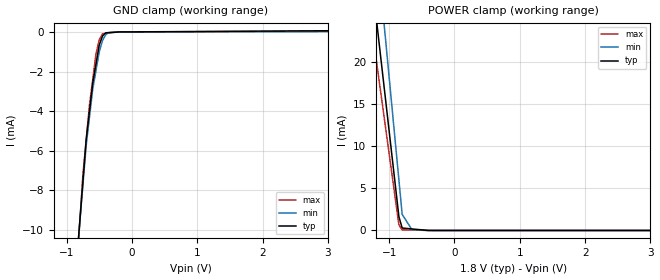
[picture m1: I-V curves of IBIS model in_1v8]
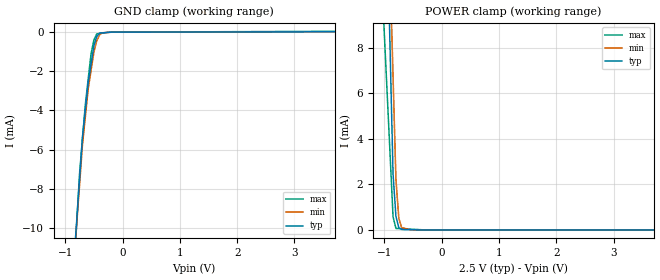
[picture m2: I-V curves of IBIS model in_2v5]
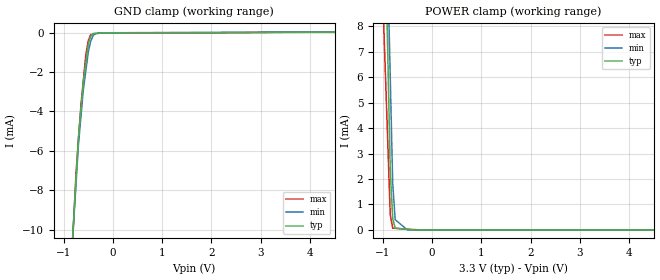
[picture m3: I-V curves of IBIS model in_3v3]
[IBIS Ver]   3.2
[Comment Char] |_char
[File Name]   tlv320aic25i.ibs
[File Rev]   3.0
[Source]
| This model file was created by Teraspeed Consulting Group LLC
| (http://www.teraspeed.com/).
[Date]   10-06-2007
[Notes]   Quality Check of this IBIS model: Model Passes IBIS Check
   Model parses into ICX IS. Simulation done with Hyperlynx.
   1. MIN TYP MAX information is based on Temprature and Voltage
   characteristics only.
[Disclaimer]
| This model is designed as an aid for customers of Texas Instruments.
| TI and its licensors and suppliers make no warranties, either expressed
| or implied, with respect to this  model, including the warranties of
| merchantability or fitness for a particular purpose.
| The model is provided solely on an "as is" basis. The entire risk as to
| its quality and performance is with the customer.
[Copyright]
| (C) Copyright 2008 Texas Instruments Incorporated. All rights reserved.
[Component] TLV320AIC25I
[Manufacturer] TI
[Package]
| variable   typ   min   max
R_pkg  1.8006E-02  1.8006E-02  1.8006E-02
L_pkg  2.1607E-09  2.1607E-09  2.1607E-09
C_pkg  6.0021E-13  6.0021E-13  6.0021E-13
[Pin] signal_name  model_name  R_pin  L_pin C_pin
1   HDSI-   analog   1.89E-02  2.26E-09  6.29E-13
2   HDSI+   analog   1.80E-02  2.16E-09  6.01E-13
3   HDSO-   analog   1.72E-02  2.06E-09  5.73E-13
4   HDSO+   analog   1.64E-02  1.97E-09  5.47E-13
5   AVDD2   POWER   1.56E-02  1.87E-09  5.21E-13
6   AVSS2   GND   1.49E-02  1.78E-09  4.96E-13
7   TESTP   analog   1.49E-02  1.78E-09  4.96E-13
8   NC   NC   1.56E-02  1.87E-09  5.21E-13
9   _PWRDN   in   1.64E-02  1.97E-09  5.47E-13
10   SDA   out_io_od 1.72E-02  2.06E-09  5.73E-13
11   SCL   in   1.80E-02  2.16E-09  6.01E-13
12   IOVDD   POWER   1.89E-02  2.26E-09  6.29E-13
13   IOVSS   GND   1.89E-02  2.26E-09  6.29E-13
14   FSD   out   1.80E-02  2.16E-09  6.01E-13
15   DVDD   POWER   1.72E-02  2.06E-09  5.73E-13
16   DVSS   GND   1.64E-02  1.97E-09  5.47E-13
17   DOUT   out   1.56E-02  1.87E-09  5.21E-13
18   DIN   in   1.49E-02  1.78E-09  4.96E-13
19   FS   out_io   1.49E-02  1.78E-09  4.96E-13
20   SCLK   out_io   1.56E-02  1.87E-09  5.21E-13
21   M/S   in   1.64E-02  1.97E-09  5.47E-13
22   MCLK   in   1.72E-02  2.06E-09  5.73E-13
23   _RESET   in   1.80E-02  2.16E-09  6.01E-13
24   VSS   GND   1.89E-02  2.26E-09  6.29E-13
25   DRVSS1   GND   1.89E-02  2.26E-09  6.29E-13
26   SPKO+   analog   1.80E-02  2.16E-09  6.01E-13
27   DRVDD   POWER   1.72E-02  2.06E-09  5.73E-13
28   SPKO-   analog   1.64E-02  1.97E-09  5.47E-13
29   DRVSS2   GND   1.56E-02  1.87E-09  5.21E-13
30   CIDI-   analog   1.49E-02  1.78E-09  4.96E-13
31   CIDI+   analog   1.49E-02  1.78E-09  4.96E-13
32   AVSS1   GND   1.56E-02  1.87E-09  5.21E-13
33   AVDD1   POWER   1.64E-02  1.97E-09  5.47E-13
34   MICI-   analog   1.72E-02  2.06E-09  5.73E-13
35   MICI+   analog   1.80E-02  2.16E-09  6.01E-13
36   MICBIAS   analog   1.89E-02  2.26E-09  6.29E-13
37   LCDAC   analog   1.89E-02  2.26E-09  6.29E-13
38   HNSO-   analog   1.80E-02  2.16E-09  6.01E-13
39   HNSO+   analog   1.72E-02  2.06E-09  5.73E-13
40   HNSI-   analog   1.64E-02  1.97E-09  5.47E-13
41   HNSI+   analog   1.56E-02  1.87E-09  5.21E-13
42   AVDD   POWER   1.49E-02  1.78E-09  4.96E-13
43   AVSS   GND   1.49E-02  1.78E-09  4.96E-13
44   LINEI+   analog   1.56E-02  1.87E-09  5.21E-13
45   LINEI-   analog   1.64E-02  1.97E-09  5.47E-13
46   LINEO-   analog   1.72E-02  2.06E-09  5.73E-13
47   LINEO+   analog   1.80E-02  2.16E-09  6.01E-13
48   NC   NC   1.89E-02  2.26E-09  6.29E-13
[Model Selector] in
in_1v8   input IOVDD=1.8V
in_2v5   input IOVDD=2.5V
in_3v3   input IOVDD=3.3V
[Model Selector] out
out_1v8  output IOVDD=1.8V
out_2v5  output IOVDD=2.5V
out_3v3  output IOVDD=3.3V
[Model Selector] out_io
io_1v8   io output IOVDD=1.8V
io_2v5   io output IOVDD=2.5V
io_3v3   io output IOVDD=3.3V
[Model Selector] out_io_od
od_1v8   open drain io IOVDD=1.8V
od_2v5   open drain io IOVDD=2.5V
od_3v3   open drain io IOVDD=3.3V
[Model] analog
Model_type Terminator
C_comp  0pF 0pF 0pF
| variable typ   min   max
[Voltage Range]   3.30000V  3.00000V  3.60000V
[POWER Clamp Reference]  3.30000V  3.00000V  3.60000V
[GND Clamp Reference]   0.00000V  0.00000V  0.00000V
[Temperature Range]   25   85   -40
| Models and submodels in the file (13): analog (Terminator), in_1v8 (Input), in_2v5 (Input), in_3v3 (Input), io_1v8 (I/O), io_2v5 (I/O), io_3v3 (I/O), od_1v8 (I/O_open_drain), od_2v5 (I/O_open_drain), od_3v3 (I/O_open_drain), out_1v8 (Output), out_2v5 (Output), out_3v3 (Output)
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[Model] in_1v8
Model_type Input
Vinl = 540.000mV
Vinh = 1.26000V
C_comp 865.00fF 865.00fF 865.00fF
| variable typ   min   max
[Voltage Range] 1.80000V 1.65000V 1.95000V
[POWER Clamp Reference] 1.80000V 1.65000V 1.95000V
[GND Clamp Reference] 0.00000V 0.00000V 0.00000V
[Temperature Range]   25   85   -40
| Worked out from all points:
|   GND clamp passes 1 mA (typ) near -0.52 V on its own axis
|   POWER clamp passes 1 mA (typ) near -0.83 V on its own axis
[GND Clamp]
-1.8V     -51.84mA   -49.48mA   -60.21mA
-750mV    -7.544mA   -7.715mA   -7.191mA
-700mV    -5.435mA   -5.726mA   -5.445mA
-650mV    -4.01mA    -4.308mA   -3.7mA
-600mV    -2.585mA   -2.89mA    -2.403mA
-550mV    -1.618mA   -1.944mA   -1.105mA
-500mV    -651.4uA   -998.2uA   -396.8uA
-450mV    -202.3uA   -430uA     -89.27uA
-400mV    -42.24uA   -132.6uA   -69.57uA
-350mV    -31.55uA   -30.96uA   -49.87uA
-175mV    1.006uA    -1.033uA   -9.754nA
3.6V      72.76uA    21.19uA    45.99uA
[POWER Clamp]
-1.8V     66.17mA    83.43mA    54.33mA
-1V       11.83mA    18.22mA    9.136mA
-950mV    8.432mA    14.15mA    6.311mA
-850mV    1.64mA     5.994mA    661.3uA
-800mV    291.4uA    1.919mA    76.17uA
-650mV    182.1uA    82.36uA    52.12uA
-600mV    145.7uA    64.06uA    44.1uA
-550mV    109.3uA    45.76uA    36.08uA
-475mV    54.63uA    22.88uA    24.05uA
-400mV    0A         0A         12.03uA
-275mV    0A         0A         0A
3.6V      0A         0A         0A
[Model] in_2v5
Model_type Input
Vinl = 750.000mV
Vinh = 1.75000V
C_comp 865.00fF 865.00fF 865.00fF
| variable typ   min   max
[Voltage Range] 2.50000V 2.25000V 2.75000V
[POWER Clamp Reference] 2.50000V 2.25000V 2.75000V
[GND Clamp Reference] 0.00000V 0.00000V 0.00000V
[Temperature Range]   25   85   -40
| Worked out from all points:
|   GND clamp passes 1 mA (typ) near -0.52 V on its own axis
|   POWER clamp passes 1 mA (typ) near -0.81 V on its own axis
[GND Clamp]
-2.5V     -81.75mA   -78.51mA   -95.22mA
-750mV    -7.485mA   -7.776mA   -7.19mA
-700mV    -5.363mA   -5.755mA   -5.442mA
-650mV    -3.969mA   -4.33mA    -3.694mA
-600mV    -2.576mA   -2.904mA   -2.397mA
-550mV    -1.626mA   -1.958mA   -1.1mA
-500mV    -676.1uA   -1.011mA   -393.6uA
-450mV    -219uA     -439.1uA   -88.29uA
-400mV    -47.76uA   -136.8uA   -68.84uA
-350mV    -36.13uA   -32.34uA   -49.39uA
-175mV    -1.107uA   -1.209uA   -232.2nA
5V        25.05uA    25.91uA    55.27uA
[POWER Clamp]
-2.5V     176.6mA    155mA      87.56mA
-1.05V    23.55mA    24.69mA    11.12mA
-850mV    2.446mA    6.718mA    573.1uA
-800mV    592.9uA    2.224mA    67.58uA
-750mV    103.1uA    517.3uA    61.15uA
-700mV    22.08uA    104.5uA    54.71uA
-550mV    12.62uA    10.89uA    35.4uA
-200mV    0A         0A         0A
5V        0A         0A         0A
[Model] in_3v3
Model_type Input
Vinl = 990.000mV
Vinh = 2.31000V
C_comp 865.00fF 865.00fF 865.00fF
| variable typ   min   max
[Voltage Range] 3.30000V 3.00000V 3.60000V
[POWER Clamp Reference] 3.30000V 3.00000V 3.60000V
[GND Clamp Reference] 0.00000V 0.00000V 0.00000V
[Temperature Range]   25   85   -40
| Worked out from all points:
|   GND clamp passes 1 mA (typ) near -0.52 V on its own axis
|   POWER clamp passes 1 mA (typ) near -0.81 V on its own axis
[GND Clamp]
-3.3V     -117.1mA   -110.4mA   -136.1mA
-750mV    -7.458mA   -7.71mA    -7.174mA
-700mV    -5.309mA   -5.696mA   -5.434mA
-650mV    -3.884mA   -4.286mA   -3.693mA
-600mV    -2.46mA    -2.876mA   -2.4mA
-550mV    -1.522mA   -1.931mA   -1.106mA
-500mV    -583uA     -986.8uA   -398.9uA
-450mV    -174uA     -421.8uA   -90.18uA
-400mV    -35.63uA   -128.7uA   -70.3uA
-350mV    -26.99uA   -29.92uA   -50.41uA
-175mV    -1.051uA   -656.6nA   -701.8nA
6.6V      61.64uA    70.47uA    89.11uA
[POWER Clamp]
-3.3V     226.6mA    210.1mA    138.5mA
-1.1V     25.2mA     26.83mA    14.67mA
-850mV    2.316mA    6.004mA    595.1uA
-800mV    453.8uA    1.839mA    71.68uA
-750mV    70.63uA    403uA      65.16uA
-500mV    23.54uA    0A         32.58uA
-200mV    0A         0A         0A
6.6V      0A         0A         0A
